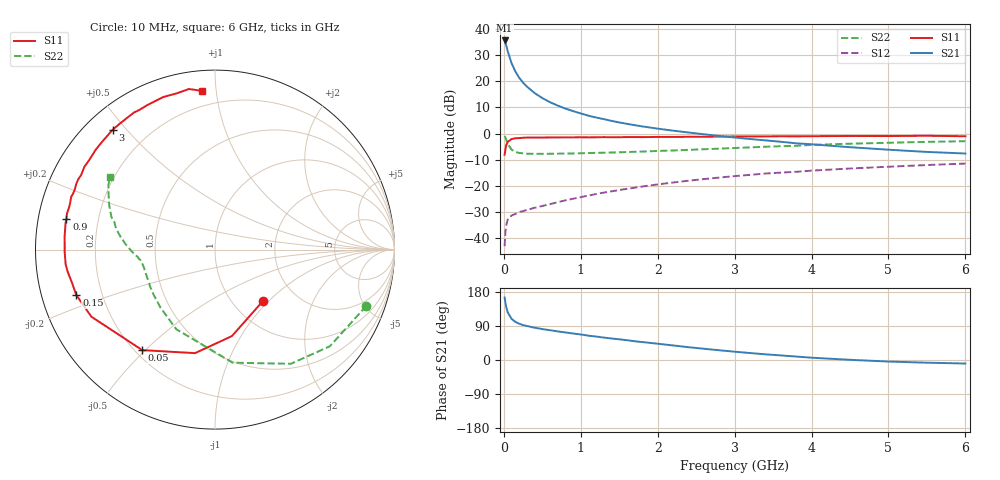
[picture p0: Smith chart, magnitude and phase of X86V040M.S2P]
! SIEMENS Small Signal Semiconductors
! BFP136W
! Si NPN RF Bipolar Junction Transistor in SOT343
! VCE = 6 V  IC = 40 mA
! Common Emitter S-Parameters:  September  1994
# GHz  S  MA  R  50
!  f  S11  S21  S12  S22
! GHz  MAG  ANG  MAG  ANG  MAG  ANG  MAG  ANG
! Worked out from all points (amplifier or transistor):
!   40 points, 10 MHz to 6 GHz, reference 50 ohm
!   highest |S21| = 35.7 dB at 10 MHz (marker M1)
!   |S21| within 3 dB of that: start of sweep to 40.48 MHz
!   unconditionally stable (mu >= 1): 793.8 MHz to 2.878 GHz
!   at 200 MHz: K = 0.48, MSG = 25.8 dB, |S12| = -30.1 dB
!   at 1.5 GHz: K = 1.12, MAG = 10.8 dB, |S12| = -21.7 dB
!   at 6 GHz: K = 0.96, MSG = 1.9 dB, |S12| = -11.5 dB
!   S11 on the Smith chart (normalised r, x): 10 MHz: 1.37, -0.93; 50 MHz: 0.23, -0.49; 150 MHz: 0.11, -0.16; 900 MHz: 0.08, +0.10; 3 GHz: 0.08, +0.46; 6 GHz: 0.11, +0.91
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0.01  0.3918 -47.1  61.17 165.0  0.0069 74.1  0.9 -20.4
0.02  0.4909 -78.9  55.39 151.6  0.0127 64.7  0.8363 -40.1
0.03  0.5875 -100.9  49.7 140.9  0.0171 55.3  0.7638 -56.4
0.05  0.6913 -125.9  38.21 125.9  0.0223 42.5  0.6379 -81.1
0.1  0.7836 -151.5  22.45 108.5  0.0267 32.7  0.4932 -116.0
0.15  0.8131 -161.8  15.52 100.6  0.0287 31.7  0.443 -133.4
0.2  0.8188 -167.4  11.74 95.7  0.0311 31.9  0.4246 -143.5
0.25  0.8301 -171.5  9.496 92.2  0.0326 32.6  0.4162 -150.1
0.3  0.8362 -174.4  7.957 89.7  0.0341 34.0  0.4105 -154.6
0.4  0.8376 -179.1  6 85.2  0.0376 37.2  0.4082 -160.4
0.5  0.8383 177.4  4.791 81.6  0.0407 40.4  0.4078 -164.2
0.6  0.8411 175.1  3.999 78.7  0.0442 43.2  0.4093 -166.6
0.7  0.8426 172.3  3.445 75.4  0.0481 45.7  0.4111 -168.2
0.9  0.8456 168.3  2.694 70.0  0.0561 48.9  0.415 -170.9
1.1  0.8461 163.6  2.203 64.2  0.0645 51.3  0.4223 -172.4
1.5  0.8501 156.6  1.633 54.6  0.0824 53.6  0.4367 -175.1
2.2  0.8605 144.1  1.136 38.4  0.1149 52.2  0.4733 179.9
3  0.8783 130.4  0.841 21.9  0.1525 47.2  0.528 172.8
3.2  0.8797 127.0  0.786 18.4  0.1611 45.5  0.5421 170.7
4.5  0.8977 108.7  0.547 0.5  0.2135 34.8  0.6389 157.3
5.5  0.9064 99.2  0.444 -7.1  0.2487 26.8  0.6929 149.0
6  0.8878 94.8  0.414 -9.3  0.2656 22.4  0.7125 145.4
